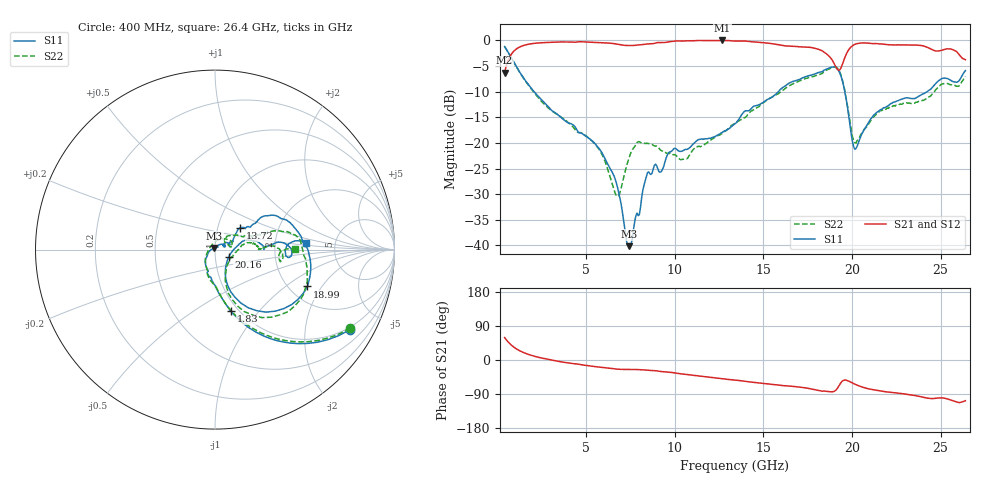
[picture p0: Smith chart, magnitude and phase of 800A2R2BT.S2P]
!  American Technical Ceramics  Date:  12/17/08
!  One Norden Lane
!  Huntington Station,  NY.  11746-2102
!  Tel:  (631) 622-4700  Fax:  (631) 622-4748
!  Part Number  800A2R2BT
!  Description: Broardband capacitor  Mounting Orientation: Vertical
!  Application:
# GHZ S DB R 50
! Freq  |S11|  S11 Ph  |S21|  S21 Ph  |S12|  S12 Ph  |S22|  S22 Ph
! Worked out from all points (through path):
!   401 points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, 400 MHz to 26.4 GHz, reference 50 ohm
!   highest |S21| = 0.00 dB at 12.69 GHz (marker M1); lowest = -6.3 dB at 400 MHz (marker M2)
!   group delay of S21, straight-line fit = 13.2 ps
!   lowest |S11| = -40.2 dB at 7.42 GHz (marker M3), VSWR 1.02, Z = 49.7 + j0.93 ohm
!   |S11| at or under -10 dB: 2.062 GHz to 15.84 GHz (13.78 GHz wide, 154 % of centre); 19.6 GHz to 24.24 GHz (4.645 GHz wide, 21.2 % of centre)
!   |S22| runs from -30.4 to -1.2 dB; largest |S21 - S12| = 0.0091
!   S11 on the Smith chart (normalised r, x): 400 MHz: 0.91, -3.40; 1.83 GHz: 0.92, -0.72; 13.72 GHz: 1.28, +0.32; 18.99 GHz: 2.49, -1.48; 20.16 GHz: 1.16, -0.10; 26.4 GHz: 3.02, +0.32
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0.4  -1.18 -30.8  -6.30 59.1  -6.33 59.2  -1.21 -30.2
1.05  -5.05 -60.0  -1.70 29.8  -1.73 29.9  -5.09 -59.0
1.83  -9.01 -75.6  -0.68 13.4  -0.71 13.6  -9.14 -75.3
4.755  -18.13 -108.8  -0.26 -12.7  -0.27 -12.5  -18.08 -108.7
5.795  -21.39 -129.2  -0.42 -18.9  -0.42 -18.7  -21.64 -130.3
6.77  -28.65 -159.2  -0.74 -24.3  -0.74 -23.9  -30.44 145.6
7.42  -40.16 107.7  -0.98 -25.0  -0.97 -24.6  -22.95 57.0
8.395  -26.56 39.9  -0.70 -26.6  -0.68 -26.3  -20.09 14.0
9.11  -25.62 17.0  -0.41 -29.8  -0.37 -29.4  -21.01 9.9
10.54  -21.35 21.8  -0.09 -37.4  -0.08 -37.3  -23.17 38.5
12.685  -17.93 32.6  0.00 -49.4  -0.01 -49.3  -18.16 38.8
13.4  -16.26 38.5  -0.11 -53.1  -0.09 -53.0  -16.18 29.7
13.725  -14.77 40.9  -0.11 -54.6  -0.09 -54.6  -15.47 25.3
17.755  -6.70 14.8  -1.41 -76.8  -1.37 -77.0  -7.07 11.4
18.21  -6.18 5.6  -1.86 -81.2  -1.82 -81.4  -6.61 8.0
18.99  -5.13 -21.8  -4.48 -82.8  -4.45 -83.0  -5.16 -26.3
19.445  -7.70 -55.7  -4.80 -56.0  -4.77 -56.2  -7.54 -60.2
19.77  -13.55 -70.5  -2.06 -54.9  -2.02 -55.1  -13.25 -72.7
20.16  -21.24 -29.4  -0.76 -63.7  -0.73 -64.0  -19.95 -36.0
22.11  -12.55 11.4  -0.85 -84.9  -0.83 -85.2  -13.06 7.8
25.49  -7.61 -5.9  -1.63 -104.4  -1.60 -104.8  -8.57 -9.7
26.4  -5.89 4.5  -3.75 -107.4  -3.73 -107.9  -7.02 0.4
